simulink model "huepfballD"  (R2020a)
settings: Solver=ode45  StartTime=0.0  StopTime=50  RelTol=1e-3  EnableMultiTasking=on

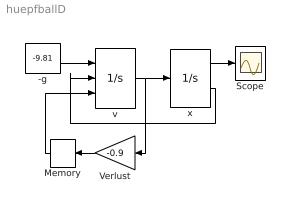
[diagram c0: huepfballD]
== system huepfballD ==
  note: .
  -g : Constant  Value=-9.81
  Memory : Memory  InitialCondition=10
  Scope : Scope
  Verlust : Gain  Gain=-0.9  SaturateOnIntegerOverflow=on
  v : Integrator  ExternalReset=falling  InitialConditionSource=external  LowerSaturationLimit=0
  x : Integrator  InitialCondition=20  LimitOutput=on  LowerSaturationLimit=0  ShowSaturationPort=on
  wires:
  v/1 -> x/1, Verlust/1
  x/1 -> Scope/1
  -g/1 -> v/1
  x/2 -> v/2
  Verlust/1 -> Memory/1
  Memory/1 -> v/3
